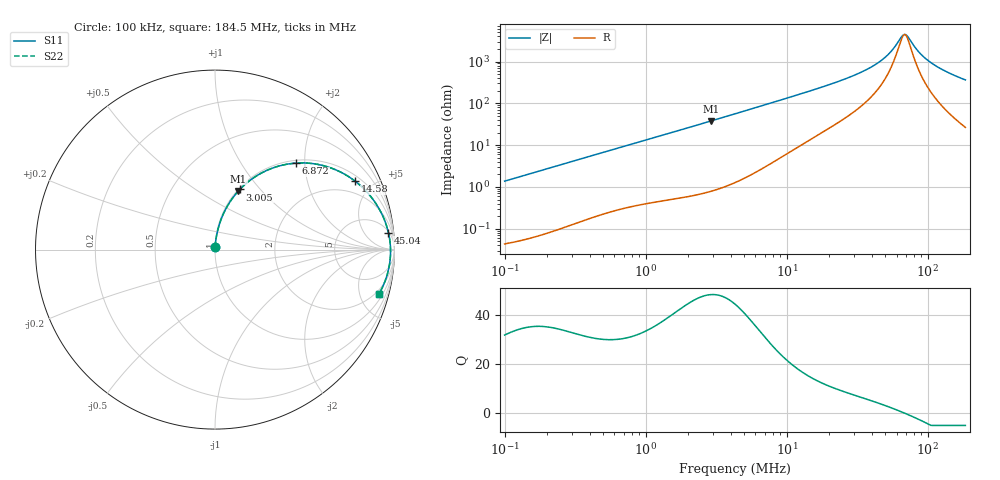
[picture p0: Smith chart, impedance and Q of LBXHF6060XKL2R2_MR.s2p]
! LBXHF6060XKL2R2_MR  S-PARAMETER MODEL  ( General Type )
! Model Generated by TAIYO YUDEN Corporation (http://www.ty-top.com)
! Version 1.0
! TAIYO YUDEN Control No. 220210
! Copyright(c) 2022 TAIYO YUDEN CO.,LTD. All Rights Reserved.
! Product Description (link to TY-COMPAS)
! https://ds.yuden.co.jp/TYCOMPAS/or/detail?pn=LBXHF6060XKL2R2NMR&u=M
! Products Name : Inductors
! Characteristics :
!  Inductance : 2.2 uH , SRF(min) : 48 MHz , DC Resistance(max) : 0.024 Ohm
!  Rated Current : Saturation :4800 mA , Temp Rise : 4700 mA
!  Case Size : 6.0 x 6.0 / 0.236 x 0.236 [mm/inch] , Thickness : 3 / 0.118 [mm/inch]
!  (Conditions: Temperature = 25 degC , DC Bias Current/Voltage = 0A / 0V)
! External Node Assignments :
!  1  o---GGG---o  2
! GND o---------o GND
! Frequency Range : 0.1MHz  -  184.468258MHz  [ 402 STEP ]
# MHz S RI R 50
! Freq[MHz].  S11 Real  S11 Imag  S21 Real  S21 Imag  S12 Real  S12 Imag  S22 Real  S22 Imag
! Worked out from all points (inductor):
!   401 points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, 100 kHz to 184.5 MHz, reference 50 ohm
!   read as one part in series: L = 2.18 uH near 103.8 kHz
!   highest Q = 48.2 at 2.894 MHz (marker M1), where L = 2.08 uH
!   self-resonance near 68.44 MHz
!   S11 on the Smith chart (normalised r, x): 100 kHz: 1.00, +0.03; 3.005 MHz: 1.02, +0.78; 6.872 MHz: 1.06, +1.81; 14.58 MHz: 1.27, +3.95; 45.04 MHz: 6, +19; 184.5 MHz: 1.53, -7.26
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0.1  0.00062 0.0137  0.9994 -0.0137  0.9994 -0.0137  0.00062 0.0137
0.352405  0.00376 0.0474  0.9962 -0.0474  0.9962 -0.0474  0.00376 0.0474
1.241892  0.03 0.1573  0.97 -0.1573  0.97 -0.1573  0.03 0.1573
1.987027  0.0678 0.2403  0.9322 -0.2403  0.9322 -0.2403  0.0678 0.2403
2.894009  0.1298 0.3259  0.8702 -0.3259  0.8702 -0.3259  0.1298 0.3259
3.004897  0.1383 0.335  0.8617 -0.335  0.8617 -0.335  0.1383 0.335
4.294977  0.2448 0.4188  0.7552 -0.4188  0.7552 -0.4188  0.2448 0.4188
6.871965  0.4519 0.482  0.5481 -0.482  0.5481 -0.482  0.4519 0.482
9.639342  0.6164 0.4644  0.3836 -0.4644  0.3836 -0.4644  0.6164 0.4644
14.57717  0.781 0.381  0.219 -0.381  0.219 -0.381  0.781 0.381
15.13571  0.793 0.3715  0.207 -0.3715  0.207 -0.3715  0.793 0.3715
29.2261  0.9295 0.1984  0.0705 -0.1984  0.0705 -0.1984  0.9295 0.1984
37.31757  0.9539 0.1384  0.0461 -0.1384  0.0461 -0.1384  0.9539 0.1384
45.03616  0.9663 0.0943  0.0337 -0.0943  0.0337 -0.0943  0.9663 0.0943
53.33896  0.9735 0.0558  0.0265 -0.0558  0.0265 -0.0558  0.9735 0.0558
65.59299  0.9778 0.00949  0.0222 -0.00949  0.0222 -0.00949  0.9778 0.00949
69.39878  0.9781 -0.00314  0.0219 0.00314  0.0219 0.00314  0.9781 -0.00314
72.05787  0.9782 -0.0116  0.0218 0.0116  0.0218 0.0116  0.9782 -0.0116
86.96199  0.976 -0.0543  0.024 0.0543  0.024 0.0543  0.976 -0.0543
102.9942  0.9704 -0.094  0.0296 0.094  0.0296 0.094  0.9704 -0.094
134.0047  0.9534 -0.1593  0.0466 0.1593  0.0466 0.1593  0.9534 -0.1593
184.4683  0.9143 -0.2457  0.0857 0.2457  0.0857 0.2457  0.9143 -0.2457
